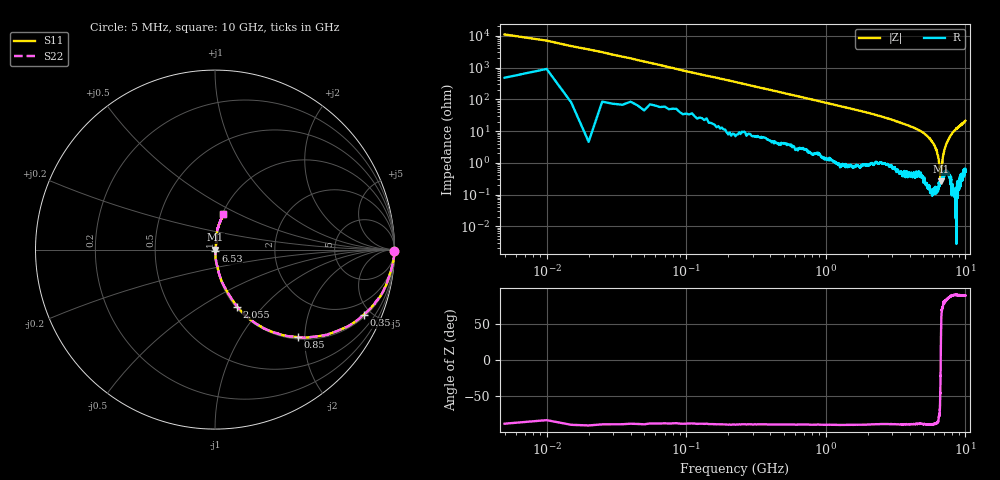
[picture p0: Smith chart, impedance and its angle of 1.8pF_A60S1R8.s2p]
! Amotech Co.,Ltd.
! http://www.amotech.co.kr/
! Part Number: A60S1R8
! These Parameters are Measured in Series Mode Connection
! Operation Temp=25[degC], DC Bias Voltage=0[V]
! Freq. Start=5[MHz] Stop=10[GHz], 2000[Steps]
! Date: Monday, July 13, 2020, 01:25:42
# GHZ S RI R 50.000000
!Freq.(Hz) S11(Real) S11(Imag) S21(Real) S21(Imag) S12(Real) S12(Imag) S22(Real) S22(Imag)
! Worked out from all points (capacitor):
!   2000 points, 5 MHz to 10 GHz, reference 50 ohm
!   read as one part in series: C = 2.06 pF near 55 MHz
!   lowest |Z| = 262 mohm at 6.65 GHz (marker M1)
!   series resonance near 6.661 GHz, so ESL is about 280 pH
!   S11 on the Smith chart (normalised r, x): 5 MHz: open; 350 MHz: 1.12, -4.51; 850 MHz: 1.04, -1.85; 2.055 GHz: 1.02, -0.73; 6.53 GHz: 1.00, -0.01; 10 GHz: 1.01, +0.42
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0.005  0.9995 -0.00903  0.000473 0.00903  0.000473 0.00903  0.9995 -0.00903
0.07  0.9873 -0.0883  0.0127 0.0883  0.0127 0.0883  0.9873 -0.0883
0.115  0.9719 -0.1447  0.0281 0.1447  0.0281 0.1447  0.9719 -0.1447
0.21  0.9303 -0.2453  0.0697 0.2453  0.0697 0.2453  0.9303 -0.2453
0.35  0.8291 -0.3632  0.1709 0.3632  0.1709 0.3632  0.8291 -0.3632
0.85  0.4611 -0.4879  0.5389 0.4879  0.5389 0.4879  0.4611 -0.4879
1.675  0.1774 -0.3731  0.8226 0.3731  0.8226 0.3731  0.1774 -0.3731
2.055  0.1239 -0.318  0.8761 0.318  0.8761 0.318  0.1239 -0.318
3.34  0.0394 -0.1816  0.9606 0.1816  0.9606 0.1816  0.0394 -0.1816
5.005  0.0101 -0.0861  0.9899 0.0861  0.9899 0.0861  0.0101 -0.0861
6.035  0.00222 -0.0342  0.9978 0.0342  0.9978 0.0342  0.00222 -0.0342
6.39  0.00181 -0.0153  0.9982 0.0153  0.9982 0.0153  0.00181 -0.0153
6.53  0.002 -0.00668  0.998 0.00668  0.998 0.00668  0.002 -0.00668
6.615  0.00259 -0.00209  0.9974 0.00209  0.9974 0.00209  0.00259 -0.00209
6.65  0.00256 -0.000519  0.9974 0.000519  0.9974 0.000519  0.00256 -0.000519
6.67  0.00291 0.000755  0.9971 -0.000755  0.9971 -0.000755  0.00291 0.000755
6.765  0.00299 0.00693  0.997 -0.00693  0.997 -0.00693  0.00299 0.00693
6.875  0.00431 0.0131  0.9957 -0.0131  0.9957 -0.0131  0.00431 0.0131
7.105  0.00546 0.0268  0.9945 -0.0268  0.9945 -0.0268  0.00546 0.0268
7.62  0.00711 0.0575  0.9929 -0.0575  0.9929 -0.0575  0.00711 0.0575
8.335  0.0112 0.1008  0.9888 -0.1008  0.9888 -0.1008  0.0112 0.1008
10  0.047 0.1992  0.953 -0.1992  0.953 -0.1992  0.047 0.1992
